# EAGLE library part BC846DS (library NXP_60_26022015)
Dual 65 V, 100 mA NPN/NPN general-purpose transistor AAL Eindhoven MK
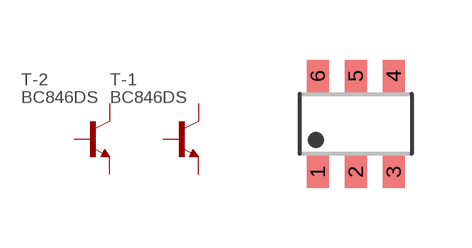
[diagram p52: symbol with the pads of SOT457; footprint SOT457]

Designator prefix T; gates -1=NPN -2=NPN

## BC846DS  [SOT457]
1  -1:E  pas
2  -1:B  pas
3  -2:C  pas
4  -2:E  pas
5  -2:B  pas
6  -1:C  pas

## Footprint SOT457 (pad centres in mm)
SOT457 TSOP6: Plastic surface-mounted package; 6 lead JEIDA: SC73 A.K.A. SOT23-6
smd 0.55 x 0.8: 1 -0.95,-1.2; 2 0,-1.2; 3 0.95,-1.2; 4 0.95,1.2; 5 0,1.2; 6 -0.95,1.2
